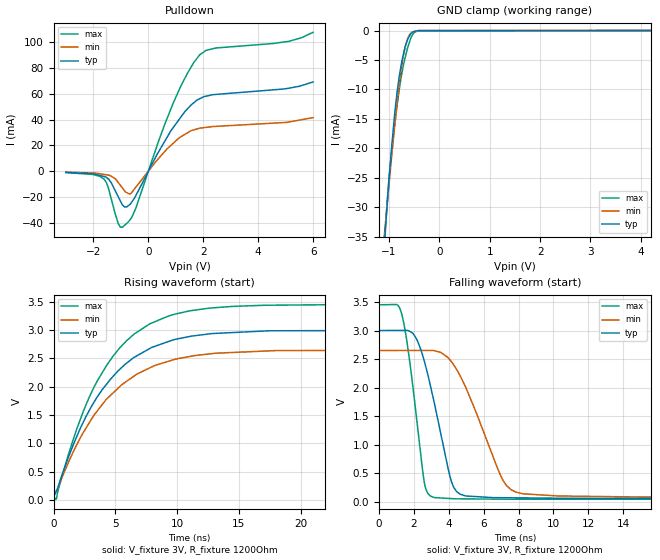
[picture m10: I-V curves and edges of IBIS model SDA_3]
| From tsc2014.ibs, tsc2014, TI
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|   3V SDA Model
[Model] SDA_3
Model_type I/O_open_drain
Polarity   Non-Inverting
Enable   Active-Low
Vinl = 0.9
Vinh = 2.1
Vmeas = 1.5
Vref = 1.5
Cref = 0pF
Rref = 50
|   typ   min   max
|   C_comp tri-state
C_comp   2.7972710e-12   2.6509420e-12   2.9513260e-12
|   C_comp high output
|C_comp   1.9121380e-11   2.2309670e-11   1.8775270e-11
|   C_comp low output
|C_comp   2.7972710e-12   2.9513260e-12   2.6509420e-12
|Where nom PVT is NOM Process, 3V,27C
|   Fast PVT is Strong Process, 3.45V, -40C
|   Slow PVT is Weak Process, 2.65V, 85C
[Model Spec]
Vinl   0.9   0.795   1.035
Vinh   2.1   1.855   2.415
| VINL 0.3 DVDD, VINH 0.7 DVDD
[Voltage Range]   3   2.65   3.45
[Temperature Range]   27   85   -40
[Pullup Reference]   3   2.65   3.45
[Pulldown Reference]   0   0   0
[Power Clamp Reference]   3   2.65   3.45
[GND Clamp Reference]   0   0   0
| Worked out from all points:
|   slope of the pulldown table from 0 to 0.45 V, typ, clamps not added: 25.1 ohm
|   GND clamp passes 1 mA (typ) near -0.60 V on its own axis
|   falling waveform, V_fixture 3V, R_fixture 1200Ohm: 20-80 % time 1.27ns typ, 2.02ns min, 814ps max; typ from 3 V to 0.058 V
|   rising waveform, V_fixture 3V, R_fixture 1200Ohm: 20-80 % time 4.87ns typ, 5.12ns min, 4.63ns max; typ from 0.058 V to 3 V
[Pulldown]
|   Voltage   I(typ)   I(min)   I(max)
-3V       -836.6uA   -613.8uA   -993.9uA
-1.62V    -4.005mA   -2.396mA   -5.909mA
-1.466V   -5.777mA   -2.925mA   -12mA
-1.093V   -19.71mA   -8.7mA     -40.47mA
-946.3mV  -25.9mA    -12.79mA   -43.26mA
-625.7mV  -24.59mA   -16.98mA   -36.49mA
877.3mV   32.99mA    21.12mA    51.24mA
1.408V    47.97mA    29.55mA    75.29mA
1.867V    56.17mA    33.34mA    90.15mA
2.45V     59.52mA    34.78mA    95.5mA
5.107V    64.35mA    38.14mA    100.6mA
6V        69.21mA    41.58mA    107.7mA
[GND Clamp]
|   Voltage   I(typ)   I(min)   I(max)
-3V       -288mA     -228.6mA   -402.1mA
-1.087V   -35.35mA   -34.19mA   -36mA
-1.072V   -33.64mA   -32.84mA   -33.98mA
-991.4mV  -24.43mA   -25.35mA   -24.21mA
-892.4mV  -14.6mA    -16.63mA   -16.31mA
-839.4mV  -10.46mA   -12.35mA   -12.7mA
-776mV    -6.751mA   -7.757mA   -8.865mA
-686.6mV  -3.008mA   -3.053mA   -4.867mA
-625.7mV  -1.422mA   -1.284mA   -2.807mA
-549.2mV  -425.9uA   -295.4uA   -976.7uA
-422.9mV  -24.35uA   -36.59uA   -31.9uA
6V        0A         0A         0A
[POWER Clamp]
|   SCR cell for ESD function. Effects occurr above VDD x 2
|   Voltage   I(typ)   I(min)   I(max)
-3V       0A         0A         0A
0V        0A         0A         0A
6V        0A         0A         0A
[Ramp]
R_load = 1200
|   typ   min   max
dV/dt_r   1.76516/4.86685e-009   1.54422/5.07067e-009   2.0437/4.62442e-009
dV/dt_f   1.76516/1.27114e-009   1.54418/2.01928e-009   2.0437/8.12058e-010
[Falling Waveform]
V_fixture = 3V
V_fixture_min = 2.65V
V_fixture_max = 3.45V
R_fixture = 1200Ohm
C_fixture = 0F
|   Time   V(typ)   V(min)   V(max)
0s        3V         2.65V      3.45V
1.294ns   3.002V     2.651V     3.301V
1.739ns   2.989V     2.651V     2.516V
2.6ns     2.464V     2.651V     339.1mV
3.171ns   1.733V     2.646V     75.63mV
4.059ns   459mV      2.49V      58.34mV
4.457ns   177.6mV    2.317V     52.91mV
7.109ns   71.99mV    376.1mV    47.03mV
8.222ns   68.78mV    142.9mV    45.5mV
50ns      58.07mV    76.36mV    43.83mV
[Rising Waveform]
V_fixture = 3V
V_fixture_min = 2.65V
V_fixture_max = 3.45V
R_fixture = 1200Ohm
C_fixture = 0F
|   Time   V(typ)   V(min)   V(max)
0s        58.07mV    76.3mV     43.83mV
237.3ps   163mV      165.9mV    20.81mV
1.238ns   774.2mV    681.4mV    827.5mV
2.447ns   1.392V     1.205V     1.586V
4.245ns   2.031V     1.769V     2.357V
6.472ns   2.51V      2.18V      2.919V
9.324ns   2.799V     2.45V      3.248V
12.5ns    2.928V     2.575V     3.383V
17.03ns   2.982V     2.628V     3.436V
50ns      3V         2.65V      3.45V
